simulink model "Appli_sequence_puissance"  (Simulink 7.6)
settings: Solver=ode15s  StartTime=0.0  StopTime=0.1  RelTol=1e-3
InitFcn:
  | clc
  | close all, clear all
  | delete *.mat
  | 
  | T=1/60; % période du signal triphasée
  | 
  | a=exp(j*2*pi/3);
  | 
  | % charge de la phase C
  | R1=2;
  | 
  | % Charge R, L de la phase B
  | R=1;
  | L=0.1;
  | 
  | % impédance interne du générateur
  | Rg=0.8929;
  | Lg=16.58e-3;
StopFcn:
  | load sequences.mat
  | 
  | plot(x(1,:),x(2,:),x(1,:),x(3,:));
  | hold on
  | 
  | plot(x(1,:),x(4,:),x(1,:),x(5,:));
  | hold on
  | 
  | plot(x(1,:),x(6,:),x(1,:),x(7,:));
  | title('Amplitudes et phases du système triphasé')
  | xlabel('temps')
  | grid
  | 
  | plot(x(1,:),x(2,:), x(1,:),x(3,:))
  | grid
  | title('Amplitude et phases des séquences pos, neg et nulle')
  | xlabel('temps')
  | grid
libraries: powerlib x6, powerlib_extras x2

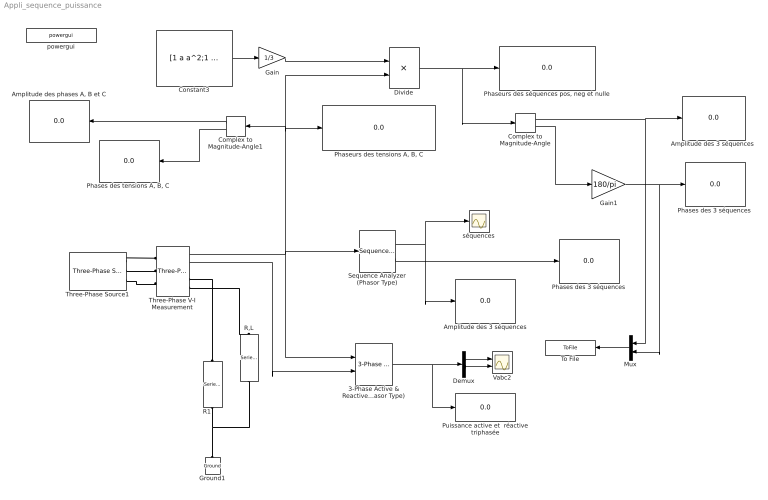
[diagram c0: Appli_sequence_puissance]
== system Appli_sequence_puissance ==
  note: F
  3-Phase Active & Reactive Power (Phasor Type) : powerlib_extras/Phasor Library/3-Phase Active & Reactive Power (Phasor Type)  DialogController=POWERSYS.PowerSysDialog  SystemSampleTime=-1
  "Amplitude des phases A, B et C" : Display
  Amplitude des 3 séquences : Display
  "Amplitude des 3 séquences " : Display
  Complex to Magnitude-Angle : ComplexToMagnitudeAngle
  Complex to Magnitude-Angle1 : ComplexToMagnitudeAngle
  Constant3 : Constant  Value=[1 a a^2;1 a^2 a; 1 1 1]
  Demux : Demux  Outputs=2
  Divide : Product  Inputs=**  Multiplication=Matrix(*)
  Gain : Gain  Gain=1/3
  Gain1 : Gain  Gain=180/pi
  Ground1 : powerlib/Elements/Ground  DialogController=POWERSYS.PowerSysDialog  PhysicalDomain=powersysdomain  SubClassName=unknown  LeftPortType=p1  RightPortType=p1  LConnTagsString=a
  Mux : Mux  Inputs=2
  Phases des 3 séquences : Display
  "Phases des 3 séquences " : Display
  "Phases des tensions A, B, C " : Display
  "Phaseurs des séquences pos, neg et nulle" : Display
  "Phaseurs des tensions A, B, C" : Display
  Puissance active et  réactive triphasée : Display
  R,L : powerlib/Elements/Series RLC Branch  DialogController=POWERSYS.PowerSysDialog  PhysicalDomain=powersysdomain  SubClassName=unknown  LeftPortType=p1  RightPortType=p1  LConnTagsString=__new0  RConnTagsString=__new0  BranchType=RL  Resistance=R  Inductance=L  SetiL0=off  InitialCurrent=0  Capacitance=1e-6  Setx0=off  InitialVoltage=0  Measurements=None
  R1 : powerlib/Elements/Series RLC Branch  DialogController=POWERSYS.PowerSysDialog  PhysicalDomain=powersysdomain  SubClassName=unknown  LeftPortType=p1  RightPortType=p1  LConnTagsString=__new0  RConnTagsString=__new0  BranchType=R  Resistance=R1  Inductance=1e-3  SetiL0=off  InitialCurrent=0  Capacitance=1e-6  Setx0=off  InitialVoltage=0  Measurements=None
  Sequence Analyzer (Phasor Type) : powerlib_extras/Phasor Library/Sequence Analyzer (Phasor Type)  DialogController=POWERSYS.PowerSysDialog  SystemSampleTime=-1  seq=Positive Negative Zero
  Three-Phase V-I Measurement : powerlib/Measurements/Three-Phase V-I Measurement  DialogController=POWERSYS.PowerSysDialog  SystemSampleTime=-1  VoltageMeasurement=phase-to-ground  SetLabelV=off  LabelV=Vabc  Vpu=off  VpuLL=off  CurrentMeasurement=yes  SetLabelI=off  LabelI=Iabc  Ipu=off  Pbase=100e6  Vbase=500e3  OutputType=Complex  PhasorSimulation=on  PSBequivalent=0
  Three-Phase Source1 : powerlib/Electrical Sources/Three-Phase Source  DialogController=POWERSYS.PowerSysDialog  SystemSampleTime=-1  Voltage=380  PhaseAngle=0  Frequency=60  InternalConnection=Yg  SpecifyImpedance=off  Resistance=Rg  Inductance=Lg  ShortCircuitLevel=100e6  BaseVoltage=25e3  XRratio=7
  To File : ToFile  Filename=sequences  MatrixName=x
  Vabc2 : Scope  NumInputPorts=2
  powergui : powerlib/powergui  Priority=1  SystemSampleTime=-1  SimulationMode=Phasor  SampleTime=50e-6  frequency=60  SPID=off  DisableSnubberDevices=off  DisableRonSwitches=off  DisableVfSwitches=off  SwTol=0  Interpol=off  frequencyindice=60  echomessages=off  HookPort=off  DisplayEquations=off  FunctionMessages=off  EnableUseOfTLC=off  x0status=blocks  RestoreLinks=warning  ResistiveCurrentMeasurement=off  Frange=[0:2:500]  Ylog=off  Xlog=on  ShowGrid=on  save=off  variable=ZData  ZoomFFT=off  StartTime=0.0  cycles=1  DisplayStyle=1  fundamental=60  FreqAxis=off  MaxFrequency=1000  frequencyindicesteady=1  display=off  methode=off
  séquences : Scope
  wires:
  Three-Phase V-I Measurement/1 -> Sequence Analyzer (Phasor Type)/1, 3-Phase Active & Reactive Power (Phasor Type)/1, "Phaseurs des tensions A, B, C"/1, Divide/2, Complex to Magnitude-Angle1/1
  Sequence Analyzer (Phasor Type)/1 -> séquences/1, Amplitude des 3 séquences/1
  Three-Phase V-I Measurement/2 -> 3-Phase Active & Reactive Power (Phasor Type)/2
  3-Phase Active & Reactive Power (Phasor Type)/1 -> Demux/1, Puissance active et  réactive triphasée/1
  Demux/1 -> Vabc2/1
  Demux/2 -> Vabc2/2
  Constant3/1 -> Gain/1
  Gain/1 -> Divide/1
  Divide/1 -> "Phaseurs des séquences pos, neg et nulle"/1, Complex to Magnitude-Angle/1
  Complex to Magnitude-Angle/1 -> "Amplitude des 3 séquences "/1, Mux/1
  Complex to Magnitude-Angle/2 -> Gain1/1
  Sequence Analyzer (Phasor Type)/2 -> Phases des 3 séquences/1
  Gain1/1 -> "Phases des 3 séquences "/1, Mux/2
  Complex to Magnitude-Angle1/1 -> "Amplitude des phases A, B et C"/1
  Complex to Magnitude-Angle1/2 -> "Phases des tensions A, B, C "/1
  Mux/1 -> To File/1
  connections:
  Three-Phase Source1/RConn1 -- Three-Phase V-I Measurement/LConn1
  Three-Phase Source1/RConn2 -- Three-Phase V-I Measurement/LConn2
  Three-Phase Source1/RConn3 -- Three-Phase V-I Measurement/LConn3
  R1/LConn1 -- Three-Phase V-I Measurement/RConn2
  Three-Phase V-I Measurement/RConn3 -- R,L/LConn1
  R,L/RConn1 -- R1/RConn1 -- Ground1/LConn1
